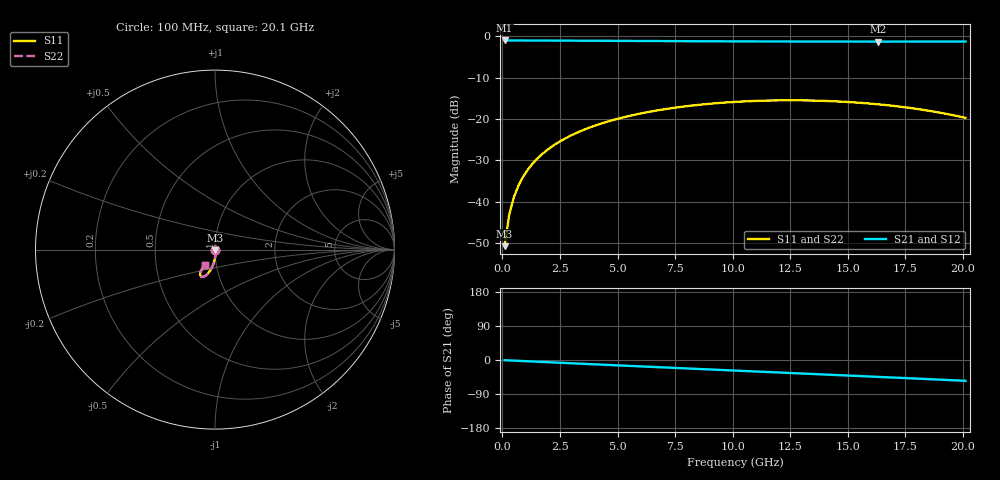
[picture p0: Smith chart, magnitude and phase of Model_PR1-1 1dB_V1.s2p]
!version-1
!date-07.2020
!Series
#GHZ S RI R 50.0
!FREQ.GHZ	S11RE	S11IM	S21RE	S21IM	S12RE	S12IM	S22RE	S22IM
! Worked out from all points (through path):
!   101 points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, 100 MHz to 20.1 GHz, reference 50 ohm
!   highest |S21| = -0.97 dB at 100 MHz (marker M1); lowest = -1.2 dB at 16.3 GHz (marker M2)
!   group delay of S21, straight-line fit = 7.51 ps
!   lowest |S11| = -50.7 dB at 100 MHz (marker M3), VSWR 1.01, Z = 50.2 - j0.219 ohm
!   |S11| at or under -10 dB: start of sweep to end of sweep
!   |S22| runs from -50.7 to -15.4 dB; largest |S21 - S12| = 0
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0.1  0.00193 -0.00218  0.894 -0.00808  0.894 -0.00808  0.00193 -0.00218
0.3  0.00224 -0.00664  0.8937 -0.017  0.8937 -0.017  0.00224 -0.00664
0.5  0.00243 -0.0111  0.8932 -0.0258  0.8932 -0.0258  0.00243 -0.0111
0.7  0.0025 -0.0155  0.8926 -0.0346  0.8926 -0.0346  0.0025 -0.0155
0.9  0.00246 -0.0199  0.8919 -0.0434  0.8919 -0.0434  0.00246 -0.0199
1.1  0.00231 -0.0243  0.8912 -0.0521  0.8912 -0.0521  0.00231 -0.0243
1.5  0.0017 -0.0329  0.8893 -0.0695  0.8893 -0.0695  0.0017 -0.0329
2.1  4.34e-05 -0.0456  0.8857 -0.0953  0.8857 -0.0953  4.34e-05 -0.0456
2.7  -0.00239 -0.0578  0.8813 -0.1208  0.8813 -0.1208  -0.00239 -0.0578
3.5  -0.00668 -0.0733  0.8742 -0.1544  0.8742 -0.1544  -0.00668 -0.0733
4.3  -0.012 -0.0877  0.8657 -0.1873  0.8657 -0.1873  -0.012 -0.0877
5.1  -0.018 -0.101  0.8559 -0.2196  0.8559 -0.2196  -0.018 -0.101
6.9  -0.0333 -0.1256  0.8297 -0.2902  0.8297 -0.2902  -0.0333 -0.1256
8.5  -0.0474 -0.1409  0.8021 -0.3503  0.8021 -0.3503  -0.0474 -0.1409
10.1  -0.0606 -0.1498  0.7707 -0.408  0.7707 -0.408  -0.0606 -0.1498
11.7  -0.0716 -0.1521  0.7359 -0.463  0.7359 -0.463  -0.0716 -0.1521
13.5  -0.0799 -0.1474  0.6929 -0.5219  0.6929 -0.5219  -0.0799 -0.1474
14.9  -0.0825 -0.1392  0.6567 -0.5655  0.6567 -0.5655  -0.0825 -0.1392
16.3  -0.0811 -0.1277  0.6179 -0.6072  0.6179 -0.6072  -0.0811 -0.1277
16.9  -0.0792 -0.122  0.6005 -0.6244  0.6005 -0.6244  -0.0792 -0.122
18.5  -0.0699 -0.1054  0.5517 -0.6688  0.5517 -0.6688  -0.0699 -0.1054
20.1  -0.0541 -0.0884  0.4989 -0.7107  0.4989 -0.7107  -0.0541 -0.0884
